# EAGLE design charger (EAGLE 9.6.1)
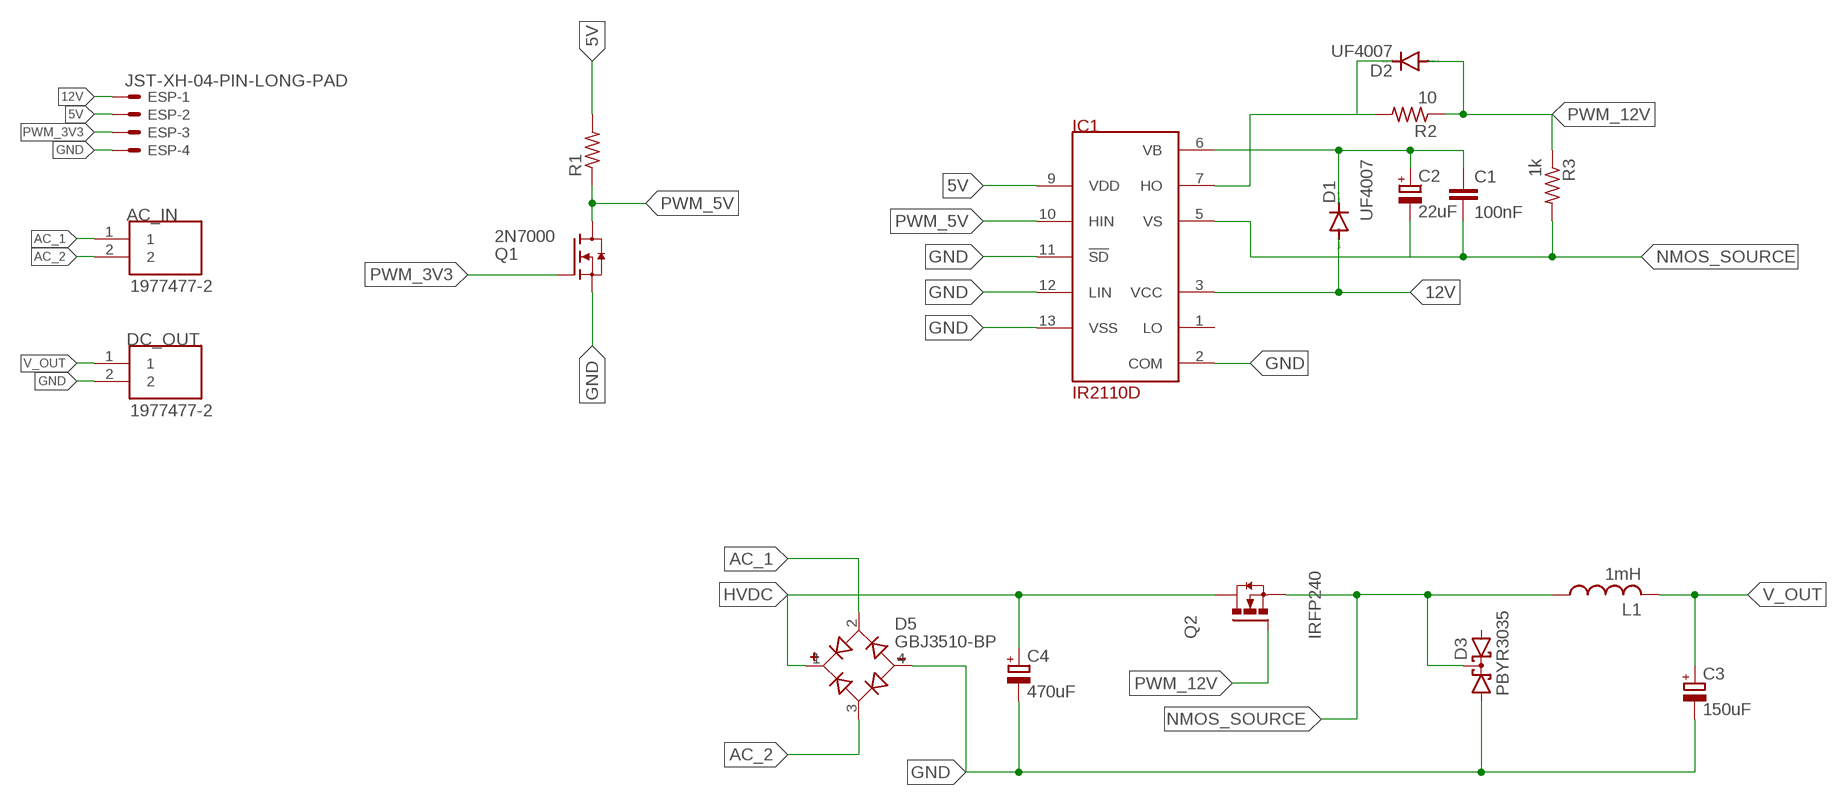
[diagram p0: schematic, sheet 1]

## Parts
AC_IN  1977477-2  [TE_1977477-2]
C1  100nF  C-EU025-025X050  [C025-025X050]
C2  22uF  CPOL-EUE2,5-6E  [E2,5-6E]
C3  150uF  CPOL-EUE7.5-18  [E7,5-18]
C4  470uF  CPOL-EUE10-35  [EB35D]
D1  UF4007  BAS15  [DO34-7]
D2  UF4007  BAS15  [DO34-7]
D3  PBYR3035  [SOT93S]
D5  GBJ3510-BP  [DIOB_GBJ3510-BP]
DC_OUT  1977477-2  [TE_1977477-2]
ESP  JST-XH-04-PIN-LONG-PAD  [JST-XH-04-PACKAGE-LONG-PAD]
IC1  IR2110D  [DIL14]
L1  1mH  L-USTJ7-U1  [TJ7-U1]
Q1  2N7000  [TO92]
Q2  IRFP240  [TO247AC]
R1  R-US_0204/7  [0204/7]
R2  10  R-US_0204/7  [0204/7]
R3  1k  R-US_0204/7  [0204/7]

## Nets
5V: ESP.2 IC1.9(VDD) R1.2
12V: D1.A ESP.1 IC1.3(VCC)
AC_1: AC_IN.1 D5.2(AC1)
AC_2: AC_IN.2 D5.3(AC2)
GND: C3.- C4.- D3.A1 D5.4(-) DC_OUT.2 ESP.4 IC1.2(COM) IC1.11(!SD) IC1.12(LIN) IC1.13(VSS) Q1.1(S)
HVDC: C4.+ D5.1(+) Q2.2(D)
N$2: D2.C IC1.7(HO) R2.2
NMOS_SOURCE: C1.2 C2.- D3.C IC1.5(VS) L1.1 Q2.3(S) R3.2
PWM_3V3: ESP.3 Q1.2(G)
PWM_5V: IC1.10(HIN) Q1.3(D) R1.1
PWM_12V: D2.A Q2.1(G) R2.1 R3.1
V_OUT: C3.+ DC_OUT.1 L1.2
VB: C1.1 C2.+ D1.C IC1.6(VB)
Unconnected: D3.A2 IC1.1(LO)

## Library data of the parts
AC_IN DC_OUT = terminal_block:1977477-2: Check availability; AVAILABILITY: In Stock; COMMENT: 1977477-2; DESCRIPTION: Conn Barrier Strip 2 POS 8.25mm Solder ST Thru-Hole 15A/Contact Carton; MF: TE Connectivity; MP: 1977477-2; PACKAGE: None; PRICE: None; PURCHASE-URL: https://pricing.snapeda.com/search/part/1977477-2/?ref=eda
C1 = rcl:C-EU: CAPACITOR, European symbol; SPICEPREFIX: C
C2-C4 = rcl:CPOL-EU: POLARIZED CAPACITOR, European symbol; SPICEPREFIX: C
D1 D2 = diode:BAS15: DIODE
D3 = diode:PBYR3035: Dual DIODE common cathode
D5 = GBJ3510-BP:GBJ3510-BP: Diode Rectifier Bridge Single 1KV 35A 4-Pin(4+Tab) Case GBJ Bulk/Tube Check availability; AVAILABILITY: In Stock; DESCRIPTION: Bridge Rectifier Single Phase Standard 1 kV Through Hole GBJ; MF: Micro Commercial; MP: GBJ3510-BP; PACKAGE: SIP-4 Micro Commercial Co; PRICE: None; PURCHASE-URL: https://pricing.snapeda.com/search/part/GBJ3510-BP/?ref=eda
ESP = Rembrandt Electronics - JST XH Connectors v1-0:JST-XH-04-PIN: JST XH Connector 2 Pin Wire to board connector. Pitch: 2,54 mm, (0.100") Number of pins: 4 Created by Rembrandt Electronics www.rembrandtelectronics.com
IC1 = irs:IR2110
L1 = custom_inductor:L-US: INDUCTOR, American symbol; SPICEPREFIX: L
Q1 = 2N7000:2N7000: Check prices; AVAILABILITY: In Stock; DESCRIPTION: N-Channel 60V 350mA (Tc) 1W (Tc) Through Hole TO-92-3; MF: STMicroelectronics; MP: 2N7000; PACKAGE: E-PKG AXIAL-LEADED-2 ON Semiconductor; PRICE: None
Q2 = IRFP240(TO-247):IRFP240: MOSFET N-CH 200V 20A TO-247AC Check availability; AVAILABILITY: In Stock; DESCRIPTION: N-Channel 200 V 20A (Tc) 150W (Tc) Through Hole TO-247AC; MF: Vishay Siliconix; MP: IRFP240; PACKAGE: TO-247 Vishay Siliconix; PRICE: None
R1-R3 = rcl:R-US_: RESISTOR, American symbol; SPICEPREFIX: R

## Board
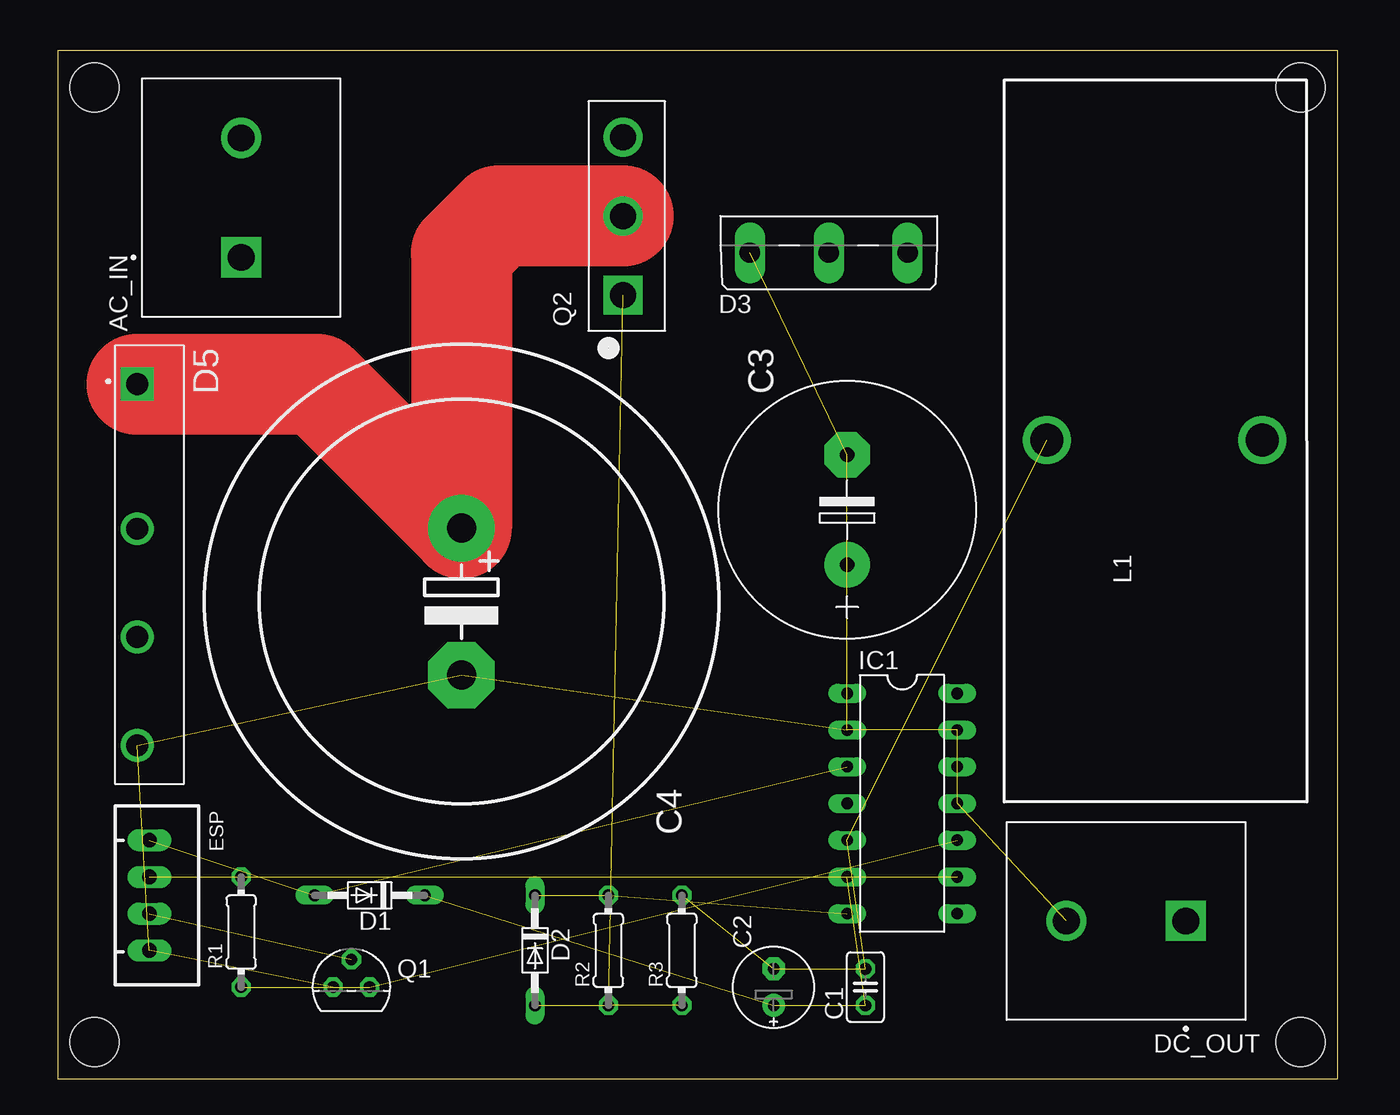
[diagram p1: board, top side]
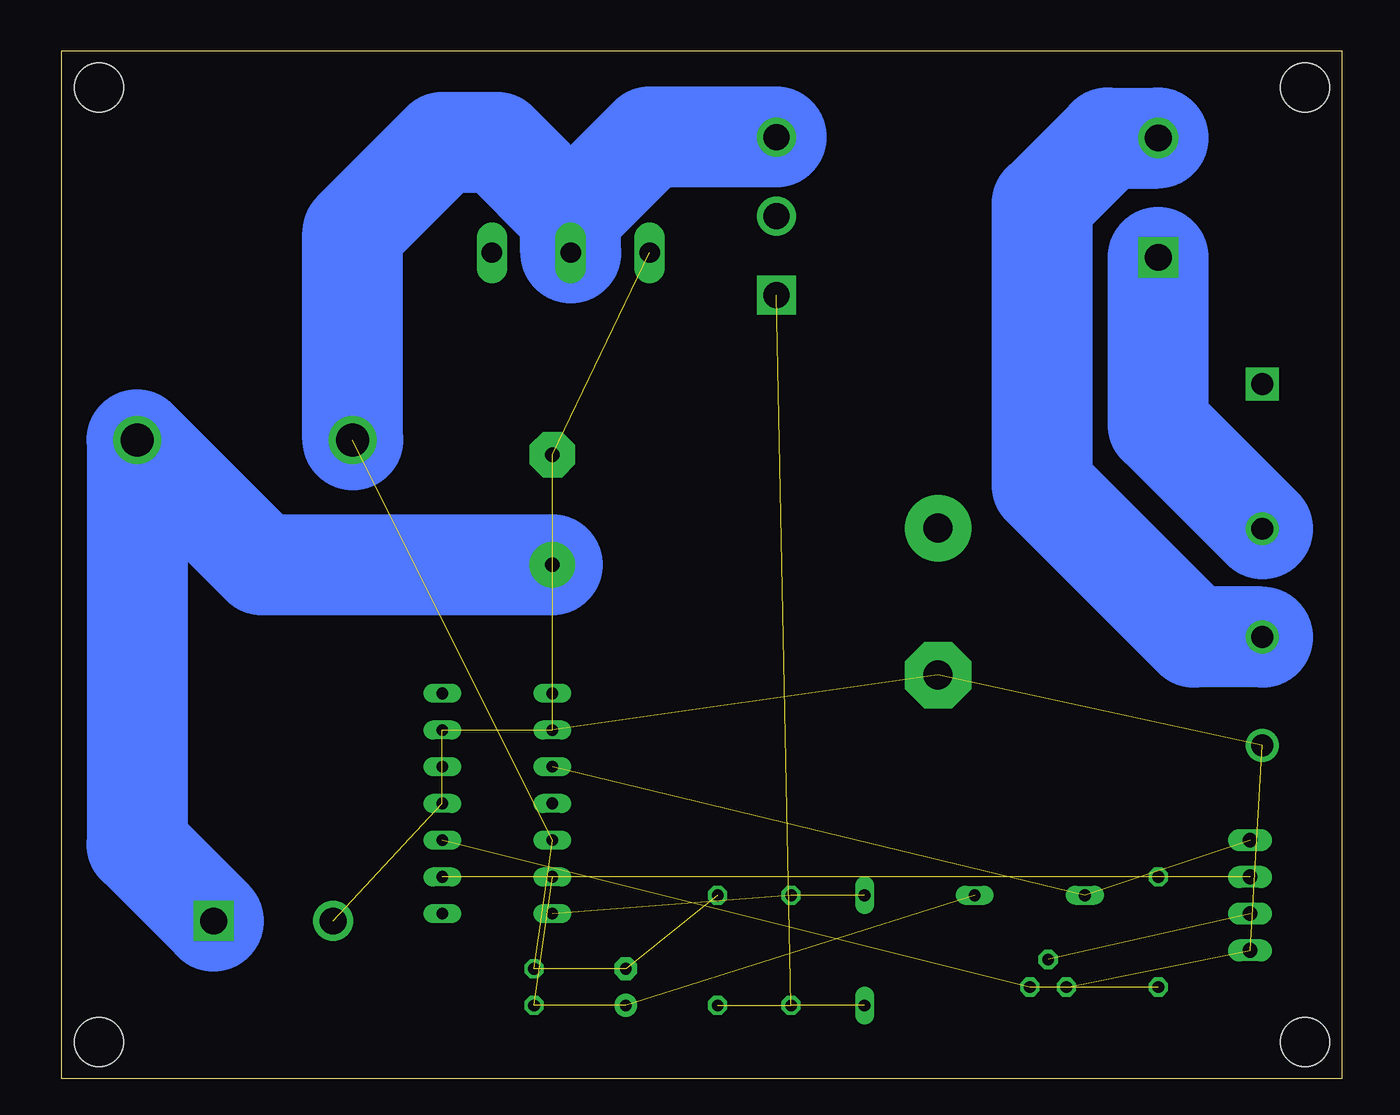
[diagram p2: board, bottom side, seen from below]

Size 88.57 x 71.11 mm. Coordinates in mm from the lower left corner, seen from the top.
Outline: 0,0 88.57,0 88.57,71.11 0,71.11 0,0
Copper layers (1*16): Top 0.035mm / dielectric 1.5mm / Bottom 0.035mm
Design rules "default *": minimum track width 12mil, minimum drill 0.35mm, track to track 12mil, track to pad 12mil, pad to pad 12mil, via to via 12mil, smd to smd 12mil, copper to edge 40mil, drill to drill 6mil, minimum pad ring 10mil, minimum via ring 8mil, stop-mask expansion 4mil, vias tented up to drill 0mil, thermal gap 10mil
Holes 3.4 mm at 2.54,68.58 85.98,68.58 2.54,2.54 85.98,2.54

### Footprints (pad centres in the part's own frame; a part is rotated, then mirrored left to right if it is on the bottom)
TE_1977477-2 = drill 1.85 square: 1 -4.13,0 | drill 1.85: 2 4.13,0
C025-025X050 = drill 0.813 octagon: 1 -1.27,0; 2 1.27,0
E2,5-6E = drill 0.813 pad 1.575: + -1.27,0 | drill 0.813 pad 1.575 octagon: - 1.27,0
E7,5-18 = drill 1.016 pad 3.15: + -3.81,0 | drill 1.016 pad 3.15 octagon: - 3.81,0
EB35D = drill 2.007 pad 4.597: + -5.08,0 | drill 2.007 pad 4.597 octagon: - 5.08,0
DO34-7 = drill 0.813 long: A 3.81,0; C -3.81,0
SOT93S = drill 1.397 long: A1 -5.461,-2.54; A2 5.461,-2.54; C 0,-2.54
DIOB_GBJ3510-BP = drill 1.51 pad 2.27 square: 1 -12.5,-0.85 | drill 1.51 pad 2.27: 2 -2.5,-0.85; 3 5,-0.85; 4 12.5,-0.85
JST-XH-04-PACKAGE-LONG-PAD = drill 1.016 long: 1 -3.81,0; 2 -1.27,0; 3 1.27,0; 4 3.81,0
DIL14 = drill 0.813 long: 1 -7.62,-3.81; 2 -5.08,-3.81; 3 -2.54,-3.81; 4 0,-3.81; 5 2.54,-3.81; 6 5.08,-3.81; 7 7.62,-3.81; 8 7.62,3.81; 9 5.08,3.81; 10 2.54,3.81; 11 0,3.81; 12 -2.54,3.81; 13 -5.08,3.81; 14 -7.62,3.81
TJ7-U1 = drill 2.286: 1 -6.503,4.826; 2 8.408,4.826
TO92 = drill 0.813 octagon: 1 -1.27,0; 2 0,1.905; 3 1.27,0
TO247AC = drill 1.79 pad 2.69 square: 1 -5.46,0.255 | drill 1.79 pad 2.69: 2 0,0.255; 3 5.46,0.255
0204/7 = drill 0.813 octagon: 1 -3.81,0; 2 3.81,0

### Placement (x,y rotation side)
AC_IN  12.7,60.96 90 top
C1  55.88,6.35 90 top
C2  49.53,6.35 90 top
C3  54.61,39.37 90 top
C4  27.94,33.02 270 top
D1  21.59,12.7 180 top
D2  33.02,8.89 270 top
D3  53.34,59.69 0 top
D5  6.35,35.56 270 top
DC_OUT  73.91,10.92 180 top
ESP  6.35,12.7 270 top
IC1  58.42,19.05 270 top
L1  74.93,39.37 0 top
Q1  20.32,6.35 0 top
Q2  39.37,59.69 90 top
R1  12.7,10.16 90 top
R2  38.1,8.89 90 top
R3  43.18,8.89 90 top

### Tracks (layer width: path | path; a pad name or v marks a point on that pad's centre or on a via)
5V  (2 unrouted)
12V  (2 unrouted)
AC_1
  Bottom 6.985: D5.2 12.7,45.26 AC_IN.1
AC_2
  Bottom 6.985: D5.3 10.24,30.56 20.73,41.05 20.73,60.55 16.19,65.09 AC_IN.2
GND  (10 unrouted)
HVDC
  Top 6.985: Q2.2 30.48,59.69 27.94,57.15 C4.+ 17.98,48.06 D5.1
N$2  (2 unrouted)
NMOS_SOURCE  (4 unrouted)
  Bottom 6.985: Q2.3 47.88,65.15 53.34,59.69 | L1.1 68.43,58.57 62.23,64.77 58.42,64.77 53.34,59.69 | D3.C 53.34,59.69
PWM_3V3  (1 unrouted)
PWM_5V  (2 unrouted)
PWM_12V  (3 unrouted)
V_OUT
  Bottom 6.985: DC_OUT.1 83.34,16.22 L1.2 74.7,35.56 C3.+
VB  (3 unrouted)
